PROGRAM Temp
VAR
	H_LID				:ARRAY[1..10] OF Temp_controller;
	H_CHAMBER			:ARRAY[1..10] OF Temp_controller;
	H_PEN_VALVE			:Temp_controller;
	H_GATE_VALVE		:Temp_controller;
	H_IGS				:ARRAY[1..10] OF Temp_controller;
	H_TAPE				:ARRAY[1..10] OF Temp_controller;
	H_FORELINE			:ARRAY[1..20] OF Temp_controller;	
END_VAR

//E01 PEN_VALVE PID		
	IF 	GV.AI.APC_Temp-GV.AO.APC_Temp_SV<3	
	THEN 
		H_PEN_VALVE.PID_Feedforward:=GV_H.PEN_VALVE_HEATER_PID.Feedforward;
	ELSE
		H_PEN_VALVE.PID_Feedforward:=0;
	END_IF	
	H_PEN_VALVE(
		ENABLE:= GV.AI.APC_Temp<110, 
		AUTO_TUNE:= GV.PEN_VALVE_HEATER_AUTO_TUNE_EN, 
		AUTO_TUNE_OUTPUT:=GV.PEN_VALVE_HEATER_AUTO_TUNE_OUTPUT,
		TEMP_SV:= GV.AO.APC_Temp_SV, 
		TEMP_ACTUAL:= GV.AI.APC_Temp, 
		TEMP_RATE:=5,
		PID_P:= GV_H.PEN_VALVE_HEATER_PID.P, 
		PID_I:= GV_H.PEN_VALVE_HEATER_PID.I, 
		PID_D:= GV_H.PEN_VALVE_HEATER_PID.D, 
		PID_Dp:= GV_H.PEN_VALVE_HEATER_PID.DP,
		PID_Output_Limit:= GV_H.PEN_VALVE_HEATER_PID.Output_Limit,
		SSR_ON=> GV.PEN_VALVE_HEATER_SSR_ON
	);		
	IF H_PEN_VALVE.PID_AUTO_TUNE_DONE
		THEN
		GV_H.PEN_VALVE_HEATER_PID.P:=H_PEN_VALVE.PID_AUTO_TUNE_P;
		GV_H.PEN_VALVE_HEATER_PID.I:=H_PEN_VALVE.PID_AUTO_TUNE_I;
		GV_H.PEN_VALVE_HEATER_PID.D:=H_PEN_VALVE.PID_AUTO_TUNE_D;
		GV.PEN_VALVE_HEATER_AUTO_TUNE_EN:=FALSE;
	END_IF
	
//E02 LID1 PID
	H_LID[1](
	ENABLE:= GV.AI.Lid_Temp<100, 
	AUTO_TUNE:= GV.LID_HEATER_AUTO_TUNE_EN[1], 
	AUTO_TUNE_OUTPUT:=GV.LID_HEATER_AUTO_TUNE_OUTPUT[1],
	TEMP_SV:= GV.AO.LID_Temp_SV, 
	TEMP_ACTUAL:= GV.AI.Lid_Temp, 
	TEMP_RATE:=5,
	PID_P:= GV_H.LID_HEATER_PID[1].P, 
	PID_I:= GV_H.LID_HEATER_PID[1].I, 
	PID_D:= GV_H.LID_HEATER_PID[1].D, 
	PID_Dp:= GV_H.LID_HEATER_PID[1].DP, 
	PID_Feedforward:= GV_H.LID_HEATER_PID[1].Feedforward,
	PID_Output_Limit:= GV_H.LID_HEATER_PID[1].Output_Limit,
	SSR_ON=> GV.LID_HEATER_SSR_ON[1],
	SSR_ON=> GV.LID_HEATER_SSR_ON[2],
	SSR_ON=> GV.LID_HEATER_SSR_ON[3],
	SSR_ON=> GV.LID_HEATER_SSR_ON[4]
	);	
	IF H_LID[1].PID_AUTO_TUNE_DONE
		THEN
		GV_H.LID_HEATER_PID[1].P:=H_LID[1].PID_AUTO_TUNE_P;
		GV_H.LID_HEATER_PID[1].I:=H_LID[1].PID_AUTO_TUNE_I;
		GV_H.LID_HEATER_PID[1].D:=H_LID[1].PID_AUTO_TUNE_D;
		GV.LID_HEATER_AUTO_TUNE_EN[1]:=FALSE;
	END_IF
//E06 CHAMBER1 PID
	H_CHAMBER[1](
	ENABLE:= GV.AI.CHAMBER_Temp1<100, 
	AUTO_TUNE:= GV.CHAMBER_HEATER_AUTO_TUNE_EN[1], 
	AUTO_TUNE_OUTPUT:=GV.CHAMBER_HEATER_AUTO_TUNE_OUTPUT[1],
	TEMP_SV:= GV.AO.Chamber_Temp1_SV, 
	TEMP_ACTUAL:= GV.AI.CHAMBER_Temp1, 
	TEMP_RATE:=5,
	PID_P:= GV_H.CHAMBER_HEATER_PID[1].P, 
	PID_I:= GV_H.CHAMBER_HEATER_PID[1].I, 
	PID_D:= GV_H.CHAMBER_HEATER_PID[1].D, 
	PID_Dp:= GV_H.CHAMBER_HEATER_PID[1].DP, 
	PID_Feedforward:= GV_H.CHAMBER_HEATER_PID[1].Feedforward,
	PID_Output_Limit:= GV_H.CHAMBER_HEATER_PID[1].Output_Limit,
	SSR_ON=> GV.CHAMBER_HEATER_SSR_ON[1],
	SSR_ON=> GV.CHAMBER_HEATER_SSR_ON[2]
	);	
	IF H_CHAMBER[1].PID_AUTO_TUNE_DONE
		THEN
		GV_H.CHAMBER_HEATER_PID[1].P:=H_CHAMBER[1].PID_AUTO_TUNE_P;
		GV_H.CHAMBER_HEATER_PID[1].I:=H_CHAMBER[1].PID_AUTO_TUNE_I;
		GV_H.CHAMBER_HEATER_PID[1].D:=H_CHAMBER[1].PID_AUTO_TUNE_D;
		GV.CHAMBER_HEATER_AUTO_TUNE_EN[1]:=FALSE;
	END_IF
//E07 CHAMBER2 PID	
	H_CHAMBER[2](
	ENABLE:= GV.AI.CHAMBER_Temp2<100, 
	AUTO_TUNE:= GV.CHAMBER_HEATER_AUTO_TUNE_EN[2], 
	AUTO_TUNE_OUTPUT:=GV.CHAMBER_HEATER_AUTO_TUNE_OUTPUT[2],
	TEMP_SV:= GV.AO.Chamber_Temp2_SV, 
	TEMP_ACTUAL:= GV.AI.CHAMBER_Temp2, 
	TEMP_RATE:=5,
	PID_P:= GV_H.CHAMBER_HEATER_PID[2].P, 
	PID_I:= GV_H.CHAMBER_HEATER_PID[2].I, 
	PID_D:= GV_H.CHAMBER_HEATER_PID[2].D, 
	PID_Dp:= GV_H.CHAMBER_HEATER_PID[2].DP, 
	PID_Feedforward:= GV_H.CHAMBER_HEATER_PID[2].Feedforward,
	PID_Output_Limit:= GV_H.CHAMBER_HEATER_PID[2].Output_Limit,
	SSR_ON=> GV.CHAMBER_HEATER_SSR_ON[3]
	);	
	IF H_CHAMBER[2].PID_AUTO_TUNE_DONE
		THEN
		GV_H.CHAMBER_HEATER_PID[2].P:=H_CHAMBER[2].PID_AUTO_TUNE_P;
		GV_H.CHAMBER_HEATER_PID[2].I:=H_CHAMBER[2].PID_AUTO_TUNE_I;
		GV_H.CHAMBER_HEATER_PID[2].D:=H_CHAMBER[2].PID_AUTO_TUNE_D;
		GV.CHAMBER_HEATER_AUTO_TUNE_EN[2]:=FALSE;
	END_IF
//E08 CHAMBER3 PID		
	H_CHAMBER[3](
	ENABLE:= GV.AI.CHAMBER_Temp3<100, 
	AUTO_TUNE:= GV.CHAMBER_HEATER_AUTO_TUNE_EN[3], 
	AUTO_TUNE_OUTPUT:=GV.CHAMBER_HEATER_AUTO_TUNE_OUTPUT[3],
	TEMP_SV:= GV.AO.Chamber_Temp3_SV, 
	TEMP_ACTUAL:= GV.AI.Chamber_Temp3, 
	TEMP_RATE:=5,
	PID_P:= GV_H.CHAMBER_HEATER_PID[3].P, 
	PID_I:= GV_H.CHAMBER_HEATER_PID[3].I, 
	PID_D:= GV_H.CHAMBER_HEATER_PID[3].D, 
	PID_Dp:= GV_H.CHAMBER_HEATER_PID[3].DP,
	PID_Feedforward:= GV_H.CHAMBER_HEATER_PID[3].Feedforward,
	PID_Output_Limit:= GV_H.CHAMBER_HEATER_PID[3].Output_Limit,
	SSR_ON=> GV.CHAMBER_HEATER_SSR_ON[4]
	);	
	IF H_CHAMBER[3].PID_AUTO_TUNE_DONE
		THEN
		GV_H.CHAMBER_HEATER_PID[3].P:=H_CHAMBER[3].PID_AUTO_TUNE_P;
		GV_H.CHAMBER_HEATER_PID[3].I:=H_CHAMBER[3].PID_AUTO_TUNE_I;
		GV_H.CHAMBER_HEATER_PID[3].D:=H_CHAMBER[3].PID_AUTO_TUNE_D;
		GV.CHAMBER_HEATER_AUTO_TUNE_EN[3]:=FALSE;
	END_IF
//E18 GATE VALVE PID
	IF 	ABS(GV.AI.GATE_VALVE_Temp-GV.AO.Gate_Valve_Temp_SV)<5	
	THEN 
		H_GATE_VALVE.PID_Feedforward:=GV_H.GATE_VALVE_HEATER_PID.Feedforward;
	ELSE
		H_GATE_VALVE.PID_Feedforward:=0;
	END_IF
	H_GATE_VALVE(
	ENABLE:= GV.AI.GATE_VALVE_Temp<100, 
	AUTO_TUNE:= GV.GATE_VALVE_HEATER_AUTO_TUNE_EN, 
	AUTO_TUNE_OUTPUT:=GV.GATE_VALVE_HEATER_AUTO_TUNE_OUTPUT,
	TEMP_SV:= GV.AO.Gate_Valve_Temp_SV, 
	TEMP_ACTUAL:= GV.AI.GATE_VALVE_Temp, 
	TEMP_RATE:=5,
	PID_P:= GV_H.GATE_VALVE_HEATER_PID.P, 
	PID_I:= GV_H.GATE_VALVE_HEATER_PID.I, 
	PID_D:= GV_H.GATE_VALVE_HEATER_PID.D, 
	PID_Dp:= GV_H.GATE_VALVE_HEATER_PID.DP, 
	PID_Output_Limit:= GV_H.GATE_VALVE_HEATER_PID.Output_Limit,
	SSR_ON=> GV.GATE_VALVE_SSR_ON
	);		
	IF H_GATE_VALVE.PID_AUTO_TUNE_DONE
		THEN
		GV_H.GATE_VALVE_HEATER_PID.P:=H_GATE_VALVE.PID_AUTO_TUNE_P;
		GV_H.GATE_VALVE_HEATER_PID.I:=H_GATE_VALVE.PID_AUTO_TUNE_I;
		GV_H.GATE_VALVE_HEATER_PID.D:=H_GATE_VALVE.PID_AUTO_TUNE_D;
		GV.GATE_VALVE_HEATER_AUTO_TUNE_EN:=FALSE;
	END_IF	
	
//E31	TAPE1 PID		
	H_TAPE[1](
	ENABLE:= GV.AI.TAPE_Temp1<120, 
	AUTO_TUNE:= GV.TAPE_HEATER_AUTO_TUNE_EN[1],
	AUTO_TUNE_OUTPUT:=GV.TAPE_HEATER_AUTO_TUNE_OUTPUT[1], 
	TEMP_SV:= GV.AO.Tape_Temp1_SV, 
	TEMP_ACTUAL:= GV.AI.TAPE_Temp1,
	TEMP_RATE:=10, 
	PID_P:= GV_H.TAPE_HEATER_PID[1].P, 
	PID_I:= GV_H.TAPE_HEATER_PID[1].I, 
	PID_D:= GV_H.TAPE_HEATER_PID[1].D, 
	PID_Dp:= GV_H.TAPE_HEATER_PID[1].DP, 
	PID_Feedforward:= GV_H.TAPE_HEATER_PID[1].Feedforward,
	PID_Output_Limit:= GV_H.TAPE_HEATER_PID[1].Output_Limit,
	SSR_ON=> GV.TAPE_HEATER_SSR_ON[1]
	);	
	IF H_TAPE[1].PID_AUTO_TUNE_DONE
		THEN
		GV_H.TAPE_HEATER_PID[1].P:=H_TAPE[1].PID_AUTO_TUNE_P;
		GV_H.TAPE_HEATER_PID[1].I:=H_TAPE[1].PID_AUTO_TUNE_I;
		GV_H.TAPE_HEATER_PID[1].D:=H_TAPE[1].PID_AUTO_TUNE_D;
		GV.TAPE_HEATER_AUTO_TUNE_EN[1]:=FALSE;
	END_IF
//E32	TAPE2 PID		
	H_TAPE[2](
	ENABLE:= GV.AI.TAPE_Temp2<120, 
	AUTO_TUNE:= GV.TAPE_HEATER_AUTO_TUNE_EN[2], 
	AUTO_TUNE_OUTPUT:=GV.TAPE_HEATER_AUTO_TUNE_OUTPUT[2], 
	TEMP_SV:= GV.AO.Tape_Temp2_SV, 
	TEMP_ACTUAL:= GV.AI.TAPE_Temp2, 
	TEMP_RATE:=10,
	PID_P:= GV_H.TAPE_HEATER_PID[2].P, 
	PID_I:= GV_H.TAPE_HEATER_PID[2].I, 
	PID_D:= GV_H.TAPE_HEATER_PID[2].D, 
	PID_Dp:= GV_H.TAPE_HEATER_PID[2].DP, 
	PID_Feedforward:= GV_H.TAPE_HEATER_PID[2].Feedforward,
	PID_Output_Limit:= GV_H.TAPE_HEATER_PID[2].Output_Limit,
	SSR_ON=> GV.TAPE_HEATER_SSR_ON[2]
	);	
	IF H_TAPE[2].PID_AUTO_TUNE_DONE
		THEN
		GV_H.TAPE_HEATER_PID[2].P:=H_TAPE[2].PID_AUTO_TUNE_P;
		GV_H.TAPE_HEATER_PID[2].I:=H_TAPE[2].PID_AUTO_TUNE_I;
		GV_H.TAPE_HEATER_PID[2].D:=H_TAPE[2].PID_AUTO_TUNE_D;
		GV.TAPE_HEATER_AUTO_TUNE_EN[2]:=FALSE;
	END_IF
//	TAPE3 PID		
	H_TAPE[3](
	ENABLE:= GV.AI.TAPE_Temp3<120, 
	AUTO_TUNE:= GV.TAPE_HEATER_AUTO_TUNE_EN[3], 
	AUTO_TUNE_OUTPUT:=GV.TAPE_HEATER_AUTO_TUNE_OUTPUT[3], 
	TEMP_SV:= GV.AO.Tape_Temp3_SV, 
	TEMP_ACTUAL:= GV.AI.TAPE_Temp3, 
	TEMP_RATE:=10,
	PID_P:= GV_H.TAPE_HEATER_PID[3].P, 
	PID_I:= GV_H.TAPE_HEATER_PID[3].I, 
	PID_D:= GV_H.TAPE_HEATER_PID[3].D, 
	PID_Dp:= GV_H.TAPE_HEATER_PID[3].DP, 
	PID_Feedforward:= GV_H.TAPE_HEATER_PID[3].Feedforward,
	PID_Output_Limit:= GV_H.TAPE_HEATER_PID[3].Output_Limit,
	SSR_ON=> GV.TAPE_HEATER_SSR_ON[3]
	);	
	IF H_TAPE[3].PID_AUTO_TUNE_DONE
		THEN
		GV_H.TAPE_HEATER_PID[3].P:=H_TAPE[3].PID_AUTO_TUNE_P;
		GV_H.TAPE_HEATER_PID[3].I:=H_TAPE[3].PID_AUTO_TUNE_I;
		GV_H.TAPE_HEATER_PID[3].D:=H_TAPE[3].PID_AUTO_TUNE_D;
		GV.TAPE_HEATER_AUTO_TUNE_EN[3]:=FALSE;
	END_IF
//E35	IGS1 PID		
	H_IGS[1](
	ENABLE:= GV.AI.IGS_Temp1<50, 
	AUTO_TUNE:= GV.IGS_HEATER_AUTO_TUNE_EN[1], 
	AUTO_TUNE_OUTPUT:=GV.IGS_HEATER_AUTO_TUNE_OUTPUT[1], 
	TEMP_SV:= GV.AO.IGS_Temp1_SV, 
	TEMP_ACTUAL:= GV.AI.IGS_Temp1, 
	TEMP_RATE:=1.5,
	PID_P:= GV_H.IGS_HEATER_PID[1].P, 
	PID_I:= GV_H.IGS_HEATER_PID[1].I, 
	PID_D:= GV_H.IGS_HEATER_PID[1].D, 
	PID_Dp:= GV_H.IGS_HEATER_PID[1].DP, 
	PID_Feedforward:= GV_H.IGS_HEATER_PID[1].Feedforward,
	PID_Output_Limit:= GV_H.IGS_HEATER_PID[1].Output_Limit,
	SSR_ON=> GV.IGS_HEATER_SSR_ON[1]
	);	
	IF H_IGS[1].PID_AUTO_TUNE_DONE
		THEN
		GV_H.IGS_HEATER_PID[1].P:=H_IGS[1].PID_AUTO_TUNE_P;
		GV_H.IGS_HEATER_PID[1].I:=H_IGS[1].PID_AUTO_TUNE_I;
		GV_H.IGS_HEATER_PID[1].D:=H_IGS[1].PID_AUTO_TUNE_D;
		GV.IGS_HEATER_AUTO_TUNE_EN[1]:=FALSE;
	END_IF
//E36	IGS2 PID	
	IF 	GV.AI.IGS_Temp2>GV.AO.IGS_Temp2_SV+3 THEN 
		H_IGS[2].PID_Feedforward:=0;
		ELSE
			H_IGS[2].PID_Feedforward:=GV_H.IGS_HEATER_PID[2].Feedforward;
	
	END_IF
	H_IGS[2](
	ENABLE:= GV.AI.IGS_Temp2<50, 
	AUTO_TUNE:= GV.IGS_HEATER_AUTO_TUNE_EN[2], 
	AUTO_TUNE_OUTPUT:=GV.IGS_HEATER_AUTO_TUNE_OUTPUT[2],
	TEMP_SV:= GV.AO.IGS_Temp2_SV, 
	TEMP_ACTUAL:= GV.AI.IGS_Temp2, 
	TEMP_RATE:=1.5,
	PID_P:= GV_H.IGS_HEATER_PID[2].P, 
	PID_I:= GV_H.IGS_HEATER_PID[2].I, 
	PID_D:= GV_H.IGS_HEATER_PID[2].D, 
	PID_Dp:= GV_H.IGS_HEATER_PID[2].DP, 
	PID_Feedforward:= GV_H.IGS_HEATER_PID[2].Feedforward,
	PID_Output_Limit:= GV_H.IGS_HEATER_PID[2].Output_Limit,
	SSR_ON=> GV.IGS_HEATER_SSR_ON[2]
	);	
	IF H_IGS[2].PID_AUTO_TUNE_DONE
		THEN
		GV_H.IGS_HEATER_PID[2].P:=H_IGS[2].PID_AUTO_TUNE_P;
		GV_H.IGS_HEATER_PID[2].I:=H_IGS[2].PID_AUTO_TUNE_I;
		GV_H.IGS_HEATER_PID[2].D:=H_IGS[2].PID_AUTO_TUNE_D;
		GV.IGS_HEATER_AUTO_TUNE_EN[2]:=FALSE;
	END_IF
//FORELINE1 PID	SSR6	AV102	
	H_FORELINE[1](
	ENABLE:= GV.AI.AV102_Temp<120, 
	AUTO_TUNE:= GV.FORELINE_HEATER_AUTO_TUNE_EN[1], 
	AUTO_TUNE_OUTPUT:=GV.FORELINE_HEATER_AUTO_TUNE_OUTPUT[1],
	TEMP_SV:= GV.AO.AV102_Temp_SV, 
	TEMP_ACTUAL:= GV.AI.AV102_Temp, 
	TEMP_RATE:=10,
	PID_P:= GV_H.FORELINE_HEATER_PID[1].P, 
	PID_I:= GV_H.FORELINE_HEATER_PID[1].I, 
	PID_D:= GV_H.FORELINE_HEATER_PID[1].D, 
	PID_Dp:= GV_H.FORELINE_HEATER_PID[1].DP, 
	PID_Feedforward:= GV_H.FORELINE_HEATER_PID[1].Feedforward,
	PID_Output_Limit:= GV_H.FORELINE_HEATER_PID[1].Output_Limit,
	SSR_ON=> GV.FORELINE_HEATER_SSR_ON[1]);
	
	IF H_FORELINE[1].PID_AUTO_TUNE_DONE
		THEN
		GV_H.FORELINE_HEATER_PID[1].P:=H_FORELINE[1].PID_AUTO_TUNE_P;
		GV_H.FORELINE_HEATER_PID[1].I:=H_FORELINE[1].PID_AUTO_TUNE_I;
		GV_H.FORELINE_HEATER_PID[1].D:=H_FORELINE[1].PID_AUTO_TUNE_D;
		GV.FORELINE_HEATER_AUTO_TUNE_EN[1]:=FALSE;
	END_IF
//FORELINE2 PID		SSR7	AV101
	H_FORELINE[2](
	ENABLE:= GV.AI.AV101_Temp<120, 
	AUTO_TUNE:= GV.FORELINE_HEATER_AUTO_TUNE_EN[2], 
	AUTO_TUNE_OUTPUT:=GV.FORELINE_HEATER_AUTO_TUNE_OUTPUT[2],
	TEMP_SV:= GV.AO.AV101_Temp_SV, 
	TEMP_ACTUAL:= GV.AI.AV101_Temp, 
	TEMP_RATE:=10,
	PID_P:= GV_H.FORELINE_HEATER_PID[2].P, 
	PID_I:= GV_H.FORELINE_HEATER_PID[2].I, 
	PID_D:= GV_H.FORELINE_HEATER_PID[2].D, 
	PID_Dp:= GV_H.FORELINE_HEATER_PID[2].DP, 
	PID_Feedforward:= GV_H.FORELINE_HEATER_PID[2].Feedforward,
	PID_Output_Limit:= GV_H.FORELINE_HEATER_PID[2].Output_Limit,
	SSR_ON=> GV.FORELINE_HEATER_SSR_ON[2]);
	
	IF H_FORELINE[2].PID_AUTO_TUNE_DONE
		THEN
		GV_H.FORELINE_HEATER_PID[2].P:=H_FORELINE[2].PID_AUTO_TUNE_P;
		GV_H.FORELINE_HEATER_PID[2].I:=H_FORELINE[2].PID_AUTO_TUNE_I;
		GV_H.FORELINE_HEATER_PID[2].D:=H_FORELINE[2].PID_AUTO_TUNE_D;
		GV.FORELINE_HEATER_AUTO_TUNE_EN[2]:=FALSE;
	END_IF
//FORELINE3 PID		SSR8	AV106
	H_FORELINE[3](
	ENABLE:= GV.AI.AV106_Temp<120, 
	AUTO_TUNE:= GV.FORELINE_HEATER_AUTO_TUNE_EN[3], 
	AUTO_TUNE_OUTPUT:=GV.FORELINE_HEATER_AUTO_TUNE_OUTPUT[3],
	TEMP_SV:= GV.AO.AV106_Temp_SV ,
	TEMP_ACTUAL:= GV.AI.AV106_Temp, 
	TEMP_RATE:=10,
	PID_P:= GV_H.FORELINE_HEATER_PID[3].P, 
	PID_I:= GV_H.FORELINE_HEATER_PID[3].I, 
	PID_D:= GV_H.FORELINE_HEATER_PID[3].D, 
	PID_Dp:= GV_H.FORELINE_HEATER_PID[3].DP, 
	PID_Feedforward:= GV_H.FORELINE_HEATER_PID[3].Feedforward,
	PID_Output_Limit:= GV_H.FORELINE_HEATER_PID[3].Output_Limit,
	SSR_ON=> GV.FORELINE_HEATER_SSR_ON[3]);
	
	IF H_FORELINE[3].PID_AUTO_TUNE_DONE
		THEN
		GV_H.FORELINE_HEATER_PID[3].P:=H_FORELINE[3].PID_AUTO_TUNE_P;
		GV_H.FORELINE_HEATER_PID[3].I:=H_FORELINE[3].PID_AUTO_TUNE_I;
		GV_H.FORELINE_HEATER_PID[3].D:=H_FORELINE[3].PID_AUTO_TUNE_D;
		GV.FORELINE_HEATER_AUTO_TUNE_EN[3]:=FALSE;
	END_IF	
//FORELINE4 PID		SSR9	BA101
	H_FORELINE[4](
	ENABLE:= GV.AI.BA01_Temp<120, 
	AUTO_TUNE:= GV.FORELINE_HEATER_AUTO_TUNE_EN[4], 
	AUTO_TUNE_OUTPUT:=GV.FORELINE_HEATER_AUTO_TUNE_OUTPUT[4],
	TEMP_SV:= GV.AO.BA01_Temp_SV, 
	TEMP_ACTUAL:= GV.AI.BA01_Temp, 
	TEMP_RATE:=10,
	PID_P:= GV_H.FORELINE_HEATER_PID[4].P, 
	PID_I:= GV_H.FORELINE_HEATER_PID[4].I, 
	PID_D:= GV_H.FORELINE_HEATER_PID[4].D, 
	PID_Dp:= GV_H.FORELINE_HEATER_PID[4].DP, 
	PID_Feedforward:= GV_H.FORELINE_HEATER_PID[4].Feedforward,
	PID_Output_Limit:= GV_H.FORELINE_HEATER_PID[4].Output_Limit,
	SSR_ON=> GV.FORELINE_HEATER_SSR_ON[4]);
	
	IF H_FORELINE[4].PID_AUTO_TUNE_DONE
		THEN
		GV_H.FORELINE_HEATER_PID[4].P:=H_FORELINE[4].PID_AUTO_TUNE_P;
		GV_H.FORELINE_HEATER_PID[4].I:=H_FORELINE[4].PID_AUTO_TUNE_I;
		GV_H.FORELINE_HEATER_PID[4].D:=H_FORELINE[4].PID_AUTO_TUNE_D;
		GV.FORELINE_HEATER_AUTO_TUNE_EN[4]:=FALSE;
	END_IF
//FORELINE5 PID		SS10	VG103
	H_FORELINE[5](
	ENABLE:= GV.AI.VG103_Pipe_Temp<120, 
	AUTO_TUNE:= GV.FORELINE_HEATER_AUTO_TUNE_EN[5], 
	TEMP_SV:= GV.AO.VG103_Pipe_Temp_SV, 
	TEMP_ACTUAL:= GV.AI.VG103_Pipe_Temp, 
	TEMP_RATE:=10,
	PID_P:= GV_H.FORELINE_HEATER_PID[5].P, 
	PID_I:= GV_H.FORELINE_HEATER_PID[5].I, 
	PID_D:= GV_H.FORELINE_HEATER_PID[5].D, 
	PID_Dp:= GV_H.FORELINE_HEATER_PID[5].DP, 
	PID_Feedforward:= GV_H.FORELINE_HEATER_PID[5].Feedforward,
	PID_Output_Limit:= GV_H.FORELINE_HEATER_PID[5].Output_Limit,
	SSR_ON=> GV.FORELINE_HEATER_SSR_ON[5]);
	
	IF H_FORELINE[5].PID_AUTO_TUNE_DONE
		THEN
		GV_H.FORELINE_HEATER_PID[5].P:=H_FORELINE[5].PID_AUTO_TUNE_P;
		GV_H.FORELINE_HEATER_PID[5].I:=H_FORELINE[5].PID_AUTO_TUNE_I;
		GV_H.FORELINE_HEATER_PID[5].D:=H_FORELINE[5].PID_AUTO_TUNE_D;
		GV.FORELINE_HEATER_AUTO_TUNE_EN[5]:=FALSE;
	END_IF
//FORELINE6 PID		SSR11	EXHAUST1-6
	H_FORELINE[6](
	ENABLE:= GV.AI.Exhaust1_6_Temp<120, 
	AUTO_TUNE:= GV.FORELINE_HEATER_AUTO_TUNE_EN[6], 
	TEMP_SV:= GV.AO.Exhaust1_6_Temp_SV, 
	TEMP_ACTUAL:= GV.AI.Exhaust1_6_Temp,
	TEMP_RATE:=10, 
	PID_P:= GV_H.FORELINE_HEATER_PID[6].P, 
	PID_I:= GV_H.FORELINE_HEATER_PID[6].I, 
	PID_D:= GV_H.FORELINE_HEATER_PID[6].D, 
	PID_Dp:= GV_H.FORELINE_HEATER_PID[6].DP, 
	PID_Feedforward:= GV_H.FORELINE_HEATER_PID[6].Feedforward,
	PID_Output_Limit:= GV_H.FORELINE_HEATER_PID[6].Output_Limit,
	SSR_ON=> GV.FORELINE_HEATER_SSR_ON[6]);
	
	IF H_FORELINE[6].PID_AUTO_TUNE_DONE
		THEN
		GV_H.FORELINE_HEATER_PID[6].P:=H_FORELINE[6].PID_AUTO_TUNE_P;
		GV_H.FORELINE_HEATER_PID[6].I:=H_FORELINE[6].PID_AUTO_TUNE_I;
		GV_H.FORELINE_HEATER_PID[6].D:=H_FORELINE[6].PID_AUTO_TUNE_D;
		GV.FORELINE_HEATER_AUTO_TUNE_EN[6]:=FALSE;
	END_IF
//FORELINE7 PID		SSR12	EXHAUST7-8
	H_FORELINE[7](
	ENABLE:= GV.AI.Exhaust7_8_Temp<120, 
	AUTO_TUNE:= GV.FORELINE_HEATER_AUTO_TUNE_EN[7], 
	TEMP_SV:= GV.AO.Exhaust7_8_Temp_SV, 
	TEMP_ACTUAL:= GV.AI.Exhaust7_8_Temp, 
	TEMP_RATE:=10,
	PID_P:= GV_H.FORELINE_HEATER_PID[7].P, 
	PID_I:= GV_H.FORELINE_HEATER_PID[7].I, 
	PID_D:= GV_H.FORELINE_HEATER_PID[7].D, 
	PID_Dp:= GV_H.FORELINE_HEATER_PID[7].DP, 
	PID_Feedforward:= GV_H.FORELINE_HEATER_PID[7].Feedforward,
	PID_Output_Limit:= GV_H.FORELINE_HEATER_PID[7].Output_Limit,
	SSR_ON=> GV.FORELINE_HEATER_SSR_ON[7]);
	
	IF H_FORELINE[7].PID_AUTO_TUNE_DONE
		THEN
		GV_H.FORELINE_HEATER_PID[7].P:=H_FORELINE[7].PID_AUTO_TUNE_P;
		GV_H.FORELINE_HEATER_PID[7].I:=H_FORELINE[7].PID_AUTO_TUNE_I;
		GV_H.FORELINE_HEATER_PID[7].D:=H_FORELINE[7].PID_AUTO_TUNE_D;
		GV.FORELINE_HEATER_AUTO_TUNE_EN[7]:=FALSE;
	END_IF
//FORELINE8 PID		SSR13
	H_FORELINE[8](
	ENABLE:= GV.AI.VG101_Pipe_Temp<120, 
	AUTO_TUNE:= GV.FORELINE_HEATER_AUTO_TUNE_EN[8], 
	TEMP_SV:= GV.AO.VG101_Pipe_Temp_SV, 
	TEMP_ACTUAL:= GV.AI.VG101_Pipe_Temp, 
	TEMP_RATE:=10,
	PID_P:= GV_H.FORELINE_HEATER_PID[8].P, 
	PID_I:= GV_H.FORELINE_HEATER_PID[8].I, 
	PID_D:= GV_H.FORELINE_HEATER_PID[8].D, 
	PID_Dp:= GV_H.FORELINE_HEATER_PID[8].DP, 
	PID_Feedforward:= GV_H.FORELINE_HEATER_PID[8].Feedforward,
	PID_Output_Limit:= GV_H.FORELINE_HEATER_PID[8].Output_Limit,
	SSR_ON=> GV.FORELINE_HEATER_SSR_ON[8]);
	
	IF H_FORELINE[8].PID_AUTO_TUNE_DONE
		THEN
		GV_H.FORELINE_HEATER_PID[8].P:=H_FORELINE[8].PID_AUTO_TUNE_P;
		GV_H.FORELINE_HEATER_PID[8].I:=H_FORELINE[8].PID_AUTO_TUNE_I;
		GV_H.FORELINE_HEATER_PID[8].D:=H_FORELINE[8].PID_AUTO_TUNE_D;
		GV.FORELINE_HEATER_AUTO_TUNE_EN[8]:=FALSE;
	END_IF
(*	//FORELINE9 PID		
	H_FORELINE[9](
	ENABLE:= GV.AI.FORELINE_Temp9<120, 
	AUTO_TUNE:= GV.FORELINE_HEATER_AUTO_TUNE_EN[9], 
	TEMP_SV:= FORELINE_TEMP_SV[9], 
	TEMP_ACTUAL:= GV.AI.FORELINE_Temp9, 
	PID_P:= GV_H.FORELINE_HEATER_PID[9].P, 
	PID_I:= GV_H.FORELINE_HEATER_PID[9].I, 
	PID_D:= GV_H.FORELINE_HEATER_PID[9].D, 
	PID_Dp:= GV_H.FORELINE_HEATER_PID[9].DP, 
	PID_Feedforward:= GV_H.FORELINE_HEATER_PID[9].Feedforward,
	PID_Output_Limit:= GV_H.FORELINE_HEATER_PID[9].Output_Limit,
	SSR_ON=> GV.FORELINE_HEATER_SSR_ON[9]);
	
	IF H_FORELINE[9].PID_AUTO_TUNE_DONE
		THEN
		GV_H.FORELINE_HEATER_PID[9].P:=H_FORELINE[9].PID_AUTO_TUNE_P;
		GV_H.FORELINE_HEATER_PID[9].I:=H_FORELINE[9].PID_AUTO_TUNE_I;
		GV_H.FORELINE_HEATER_PID[9].D:=H_FORELINE[9].PID_AUTO_TUNE_D;
		GV.FORELINE_HEATER_AUTO_TUNE_EN[9]:=FALSE;
	END_IF
	//FORELINE10 PID		
	H_FORELINE[10](
	ENABLE:= GV.AI.FORELINE_Temp10<120, 
	AUTO_TUNE:= GV.FORELINE_HEATER_AUTO_TUNE_EN[10], 
	TEMP_SV:= FORELINE_TEMP_SV[10], 
	TEMP_ACTUAL:= GV.AI.FORELINE_Temp10, 
	PID_P:= GV_H.FORELINE_HEATER_PID[10].P, 
	PID_I:= GV_H.FORELINE_HEATER_PID[10].I, 
	PID_D:= GV_H.FORELINE_HEATER_PID[10].D, 
	PID_Dp:= GV_H.FORELINE_HEATER_PID[10].DP, 
	PID_Feedforward:= GV_H.FORELINE_HEATER_PID[10].Feedforward,
	PID_Output_Limit:= GV_H.FORELINE_HEATER_PID[10].Output_Limit,
	SSR_ON=> GV.FORELINE_HEATER_SSR_ON[10]);
	
	IF H_FORELINE[10].PID_AUTO_TUNE_DONE
		THEN
		GV_H.FORELINE_HEATER_PID[10].P:=H_FORELINE[10].PID_AUTO_TUNE_P;
		GV_H.FORELINE_HEATER_PID[10].I:=H_FORELINE[10].PID_AUTO_TUNE_I;
		GV_H.FORELINE_HEATER_PID[10].D:=H_FORELINE[10].PID_AUTO_TUNE_D;
		GV.FORELINE_HEATER_AUTO_TUNE_EN[10]:=FALSE;
	END_IF
	//FORELINE11 PID		
	H_FORELINE[11](
	ENABLE:= GV.AI.FORELINE_Temp11<120, 
	AUTO_TUNE:= GV.FORELINE_HEATER_AUTO_TUNE_EN[11], 
	TEMP_SV:= FORELINE_TEMP_SV[11], 
	TEMP_ACTUAL:= GV.AI.FORELINE_Temp11, 
	PID_P:= GV_H.FORELINE_HEATER_PID[11].P, 
	PID_I:= GV_H.FORELINE_HEATER_PID[11].I, 
	PID_D:= GV_H.FORELINE_HEATER_PID[11].D, 
	PID_Dp:= GV_H.FORELINE_HEATER_PID[11].DP, 
	PID_Feedforward:= ,
	PID_Output_Limit:= GV_H.FORELINE_HEATER_PID[11].Output_Limit,
	SSR_ON=> GV.FORELINE_HEATER_SSR_ON[11]);
	
	IF H_FORELINE[11].PID_AUTO_TUNE_DONE
		THEN
		GV_H.FORELINE_HEATER_PID[11].P:=H_FORELINE[11].PID_AUTO_TUNE_P;
		GV_H.FORELINE_HEATER_PID[11].I:=H_FORELINE[11].PID_AUTO_TUNE_I;
		GV_H.FORELINE_HEATER_PID[11].D:=H_FORELINE[11].PID_AUTO_TUNE_D;
		GV.FORELINE_HEATER_AUTO_TUNE_EN[11]:=FALSE;
	END_IF
	//FORELINE12 PID		
	H_FORELINE[12](
	ENABLE:= GV.AI.FORELINE_Temp12<120, 
	AUTO_TUNE:= GV.FORELINE_HEATER_AUTO_TUNE_EN[12], 
	TEMP_SV:= FORELINE_TEMP_SV[12], 
	TEMP_ACTUAL:= GV.AI.FORELINE_Temp12, 
	PID_P:= GV_H.FORELINE_HEATER_PID[12].P, 
	PID_I:= GV_H.FORELINE_HEATER_PID[12].I, 
	PID_D:= GV_H.FORELINE_HEATER_PID[12].D, 
	PID_Dp:= GV_H.FORELINE_HEATER_PID[12].DP, 
	PID_Feedforward:= ,
	PID_Output_Limit:= GV_H.FORELINE_HEATER_PID[12].Output_Limit,
	SSR_ON=> GV.FORELINE_HEATER_SSR_ON[12]);
	
	IF H_FORELINE[12].PID_AUTO_TUNE_DONE
		THEN
		GV_H.FORELINE_HEATER_PID[12].P:=H_FORELINE[12].PID_AUTO_TUNE_P;
		GV_H.FORELINE_HEATER_PID[12].I:=H_FORELINE[12].PID_AUTO_TUNE_I;
		GV_H.FORELINE_HEATER_PID[12].D:=H_FORELINE[12].PID_AUTO_TUNE_D;
		GV.FORELINE_HEATER_AUTO_TUNE_EN[12]:=FALSE;
	END_IF
	//FORELINE13 PID		
	H_FORELINE[13](
	ENABLE:= GV.AI.FORELINE_Temp13<120, 
	AUTO_TUNE:= GV.FORELINE_HEATER_AUTO_TUNE_EN[13], 
	TEMP_SV:= FORELINE_TEMP_SV[13], 
	TEMP_ACTUAL:= GV.AI.FORELINE_Temp13, 
	PID_P:= GV_H.FORELINE_HEATER_PID[13].P, 
	PID_I:= GV_H.FORELINE_HEATER_PID[13].I, 
	PID_D:= GV_H.FORELINE_HEATER_PID[13].D, 
	PID_Dp:= GV_H.FORELINE_HEATER_PID[13].DP, 
	PID_Feedforward:= ,
	PID_Output_Limit:= GV_H.FORELINE_HEATER_PID[13].Output_Limit,
	SSR_ON=> GV.FORELINE_HEATER_SSR_ON[13]);
	
	IF H_FORELINE[13].PID_AUTO_TUNE_DONE
		THEN
		GV_H.FORELINE_HEATER_PID[13].P:=H_FORELINE[13].PID_AUTO_TUNE_P;
		GV_H.FORELINE_HEATER_PID[13].I:=H_FORELINE[13].PID_AUTO_TUNE_I;
		GV_H.FORELINE_HEATER_PID[13].D:=H_FORELINE[13].PID_AUTO_TUNE_D;
		GV.FORELINE_HEATER_AUTO_TUNE_EN[13]:=FALSE;
	END_IF
	//FORELINE14 PID		
	H_FORELINE[14](
	ENABLE:= GV.AI.FORELINE_Temp14<120, 
	AUTO_TUNE:= GV.FORELINE_HEATER_AUTO_TUNE_EN[14], 
	TEMP_SV:= FORELINE_TEMP_SV[14], 
	TEMP_ACTUAL:= GV.AI.FORELINE_Temp14, 
	PID_P:= GV_H.FORELINE_HEATER_PID[14].P, 
	PID_I:= GV_H.FORELINE_HEATER_PID[14].I, 
	PID_D:= GV_H.FORELINE_HEATER_PID[14].D, 
	PID_Dp:= GV_H.FORELINE_HEATER_PID[14].DP, 
	PID_Feedforward:= ,
	PID_Output_Limit:= GV_H.FORELINE_HEATER_PID[14].Output_Limit,
	SSR_ON=> GV.FORELINE_HEATER_SSR_ON[14]);
	
	IF H_FORELINE[14].PID_AUTO_TUNE_DONE
		THEN
		GV_H.FORELINE_HEATER_PID[14].P:=H_FORELINE[14].PID_AUTO_TUNE_P;
		GV_H.FORELINE_HEATER_PID[14].I:=H_FORELINE[14].PID_AUTO_TUNE_I;
		GV_H.FORELINE_HEATER_PID[14].D:=H_FORELINE[14].PID_AUTO_TUNE_D;
		GV.FORELINE_HEATER_AUTO_TUNE_EN[14]:=FALSE;
	END_IF
	//FORELINE15 PID		
	H_FORELINE[15](
	ENABLE:= GV.AI.FORELINE_Temp15<120, 
	AUTO_TUNE:= GV.FORELINE_HEATER_AUTO_TUNE_EN[15], 
	TEMP_SV:= FORELINE_TEMP_SV[15], 
	TEMP_ACTUAL:= GV.AI.FORELINE_Temp15, 
	PID_P:= GV_H.FORELINE_HEATER_PID[15].P, 
	PID_I:= GV_H.FORELINE_HEATER_PID[15].I, 
	PID_D:= GV_H.FORELINE_HEATER_PID[15].D, 
	PID_Dp:= GV_H.FORELINE_HEATER_PID[15].DP, 
	PID_Feedforward:= ,
	PID_Output_Limit:= GV_H.FORELINE_HEATER_PID[15].Output_Limit,
	SSR_ON=> GV.FORELINE_HEATER_SSR_ON[15]);
	
	IF H_FORELINE[15].PID_AUTO_TUNE_DONE
		THEN
		GV_H.FORELINE_HEATER_PID[15].P:=H_FORELINE[15].PID_AUTO_TUNE_P;
		GV_H.FORELINE_HEATER_PID[15].I:=H_FORELINE[15].PID_AUTO_TUNE_I;
		GV_H.FORELINE_HEATER_PID[15].D:=H_FORELINE[15].PID_AUTO_TUNE_D;
		GV.FORELINE_HEATER_AUTO_TUNE_EN[15]:=FALSE;
	END_IF
	//FORELINE16 PID		
	H_FORELINE[16](
	ENABLE:= GV.AI.FORELINE_Temp16<120, 
	AUTO_TUNE:= GV.FORELINE_HEATER_AUTO_TUNE_EN[16], 
	TEMP_SV:= FORELINE_TEMP_SV[16], 
	TEMP_ACTUAL:= GV.AI.FORELINE_Temp16, 
	PID_P:= GV_H.FORELINE_HEATER_PID[16].P, 
	PID_I:= GV_H.FORELINE_HEATER_PID[16].I, 
	PID_D:= GV_H.FORELINE_HEATER_PID[16].D, 
	PID_Dp:= GV_H.FORELINE_HEATER_PID[16].DP, 
	PID_Feedforward:= ,
	PID_Output_Limit:= GV_H.FORELINE_HEATER_PID[16].Output_Limit,
	SSR_ON=> GV.FORELINE_HEATER_SSR_ON[16]);
	
	IF H_FORELINE[16].PID_AUTO_TUNE_DONE
		THEN
		GV_H.FORELINE_HEATER_PID[16].P:=H_FORELINE[16].PID_AUTO_TUNE_P;
		GV_H.FORELINE_HEATER_PID[16].I:=H_FORELINE[16].PID_AUTO_TUNE_I;
		GV_H.FORELINE_HEATER_PID[16].D:=H_FORELINE[16].PID_AUTO_TUNE_D;
		GV.FORELINE_HEATER_AUTO_TUNE_EN[16]:=FALSE;
	END_IF
	//FORELINE17 PID		
	H_FORELINE[17](
	ENABLE:= GV.AI.FORELINE_Temp17<120, 
	AUTO_TUNE:= GV.FORELINE_HEATER_AUTO_TUNE_EN[17], 
	TEMP_SV:= FORELINE_TEMP_SV[17], 
	TEMP_ACTUAL:= GV.AI.FORELINE_Temp17, 
	PID_P:= GV_H.FORELINE_HEATER_PID[17].P, 
	PID_I:= GV_H.FORELINE_HEATER_PID[17].I, 
	PID_D:= GV_H.FORELINE_HEATER_PID[17].D, 
	PID_Dp:= GV_H.FORELINE_HEATER_PID[17].DP, 
	PID_Feedforward:= ,
	PID_Output_Limit:= GV_H.FORELINE_HEATER_PID[17].Output_Limit,
	SSR_ON=> GV.FORELINE_HEATER_SSR_ON[17]);
	
	IF H_FORELINE[17].PID_AUTO_TUNE_DONE
		THEN
		GV_H.FORELINE_HEATER_PID[17].P:=H_FORELINE[17].PID_AUTO_TUNE_P;
		GV_H.FORELINE_HEATER_PID[17].I:=H_FORELINE[17].PID_AUTO_TUNE_I;
		GV_H.FORELINE_HEATER_PID[17].D:=H_FORELINE[17].PID_AUTO_TUNE_D;
		GV.FORELINE_HEATER_AUTO_TUNE_EN[17]:=FALSE;
	END_IF
	//FORELINE18 PID		
	H_FORELINE[18](
	ENABLE:= GV.AI.FORELINE_Temp18<120, 
	AUTO_TUNE:= GV.FORELINE_HEATER_AUTO_TUNE_EN[18], 
	TEMP_SV:= FORELINE_TEMP_SV[18], 
	TEMP_ACTUAL:= GV.AI.FORELINE_Temp18, 
	PID_P:= GV_H.FORELINE_HEATER_PID[18].P, 
	PID_I:= GV_H.FORELINE_HEATER_PID[18].I, 
	PID_D:= GV_H.FORELINE_HEATER_PID[18].D, 
	PID_Dp:= GV_H.FORELINE_HEATER_PID[18].DP, 
	PID_Feedforward:= ,
	PID_Output_Limit:= GV_H.FORELINE_HEATER_PID[18].Output_Limit,
	SSR_ON=> GV.FORELINE_HEATER_SSR_ON[18]);
	
	IF H_FORELINE[18].PID_AUTO_TUNE_DONE
		THEN
		GV_H.FORELINE_HEATER_PID[18].P:=H_FORELINE[18].PID_AUTO_TUNE_P;
		GV_H.FORELINE_HEATER_PID[18].I:=H_FORELINE[18].PID_AUTO_TUNE_I;
		GV_H.FORELINE_HEATER_PID[18].D:=H_FORELINE[18].PID_AUTO_TUNE_D;
		GV.FORELINE_HEATER_AUTO_TUNE_EN[18]:=FALSE;
	END_IF
	//FORELINE19 PID		
	H_FORELINE[19](
	ENABLE:= GV.AI.FORELINE_Temp19<120, 
	AUTO_TUNE:= GV.FORELINE_HEATER_AUTO_TUNE_EN[19], 
	TEMP_SV:= FORELINE_TEMP_SV[19], 
	TEMP_ACTUAL:= GV.AI.FORELINE_Temp19, 
	PID_P:= GV_H.FORELINE_HEATER_PID[19].P, 
	PID_I:= GV_H.FORELINE_HEATER_PID[19].I, 
	PID_D:= GV_H.FORELINE_HEATER_PID[19].D, 
	PID_Dp:= GV_H.FORELINE_HEATER_PID[19].DP, 
	PID_Feedforward:= ,
	PID_Output_Limit:= GV_H.FORELINE_HEATER_PID[19].Output_Limit,
	SSR_ON=> GV.FORELINE_HEATER_SSR_ON[19]);
	
	IF H_FORELINE[19].PID_AUTO_TUNE_DONE
		THEN
		GV_H.FORELINE_HEATER_PID[19].P:=H_FORELINE[19].PID_AUTO_TUNE_P;
		GV_H.FORELINE_HEATER_PID[19].I:=H_FORELINE[19].PID_AUTO_TUNE_I;
		GV_H.FORELINE_HEATER_PID[19].D:=H_FORELINE[19].PID_AUTO_TUNE_D;
		GV.FORELINE_HEATER_AUTO_TUNE_EN[19]:=FALSE;
	END_IF
	//FORELINE20 PID		
	H_FORELINE[20](
	ENABLE:= GV.AI.FORELINE_Temp20<120, 
	AUTO_TUNE:= GV.FORELINE_HEATER_AUTO_TUNE_EN[20], 
	TEMP_SV:= FORELINE_TEMP_SV[20], 
	TEMP_ACTUAL:= GV.AI.FORELINE_Temp20, 
	PID_P:= GV_H.FORELINE_HEATER_PID[20].P, 
	PID_I:= GV_H.FORELINE_HEATER_PID[20].I, 
	PID_D:= GV_H.FORELINE_HEATER_PID[20].D, 
	PID_Dp:= GV_H.FORELINE_HEATER_PID[20].DP, 
	PID_Feedforward:= ,
	PID_Output_Limit:= GV_H.FORELINE_HEATER_PID[20].Output_Limit,
	SSR_ON=> GV.FORELINE_HEATER_SSR_ON[20]);
	
	IF H_FORELINE[20].PID_AUTO_TUNE_DONE
		THEN
		GV_H.FORELINE_HEATER_PID[20].P:=H_FORELINE[20].PID_AUTO_TUNE_P;
		GV_H.FORELINE_HEATER_PID[20].I:=H_FORELINE[20].PID_AUTO_TUNE_I;
		GV_H.FORELINE_HEATER_PID[20].D:=H_FORELINE[20].PID_AUTO_TUNE_D;
		GV.FORELINE_HEATER_AUTO_TUNE_EN[20]:=FALSE;
	END_IF
	*)

END_PROGRAM
